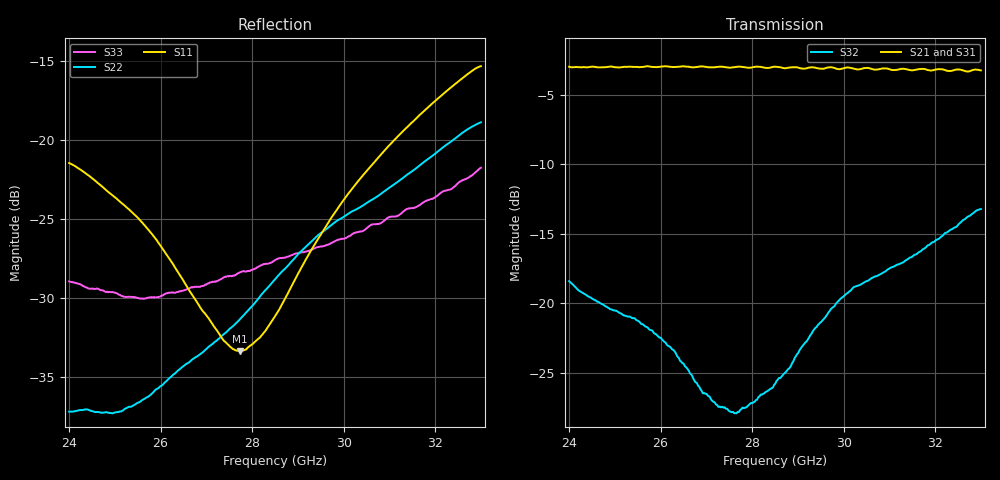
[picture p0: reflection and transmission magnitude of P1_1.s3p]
!The following data was pulled from an Agilent PNA
!This sNp file was generated from the data in the RF Test software
!NOTE:  Smoothing/Math/Corrections applied on any given trace ARE included in the data saved here
# MHz S dB R 50
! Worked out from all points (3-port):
!   1601 points, 24 GHz to 33 GHz, reference 50 ohm
!   strongest paths, dB at 24 GHz, 26.25 GHz, 28.5 GHz, 30.75 GHz, 33 GHz:
!     S21: -3.0, -3.0, -3.0, -3.2, -3.2
!     S31: -3.0, -3.0, -3.1, -3.1, -3.2
!     S32: -18.4, -23.3, -25.8, -18.0, -13.2
!   lowest |S11| = -33.4 dB at 27.73 GHz (marker M1), VSWR 1.04, Z = 50.7 + j2.03 ohm
!   |S11| at or under -10 dB: start of sweep to end of sweep
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24000  -21.47 30.3  -3.09 152.5  -3.09 153.2
       -2.98 152.6  -37.20 147.5  -18.42 104.1
       -2.98 152.8  -18.42 103.7  -28.96 -136.6
25389.38  -24.63 25.4  -3.06 138.7  -3.07 139.4
          -2.99 138.9  -36.84 142.4  -21.10 83.3
          -3.01 139.5  -21.08 83.0  -29.95 -135.6
26266.88  -27.85 26.9  -3.06 130.0  -3.07 130.7
          -3.00 129.9  -34.88 144.1  -23.34 56.8
          -2.98 130.6  -23.35 56.5  -29.68 -133.9
27234.38  -32.07 45.8  -3.06 120.1  -3.09 120.8
          -3.00 120.2  -32.68 141.2  -27.33 25.2
          -3.06 120.4  -27.33 24.9  -28.94 -138.5
27729.38  -33.37 69.1  -3.03 114.8  -3.09 115.7
          -2.98 115.0  -31.37 142.1  -27.72 6.5
          -3.11 115.8  -27.74 6.4  -28.40 -144.4
28500  -31.17 106.2  -3.07 106.8  -3.13 107.8
       -2.98 107.0  -28.83 140.4  -25.81 -33.0
       -3.12 107.9  -25.82 -33.1  -27.62 -153.4
29720.62  -24.98 127.6  -3.13 93.8  -3.17 95.1
          -3.02 94.1  -25.42 130.5  -20.43 -79.7
          -3.16 95.3  -20.43 -79.9  -26.55 -172.9
30367.5  -22.44 128.7  -3.16 86.8  -3.18 88.3
         -3.15 87.7  -24.26 124.5  -18.66 -100.1
         -3.12 88.4  -18.67 -100.2  -25.81 175.7
31678.12  -18.39 123.4  -3.24 72.6  -3.20 74.2
          -3.15 73.6  -21.59 117.1  -16.27 -122.0
          -3.18 74.7  -16.28 -122.2  -24.10 151.3
33000  -15.35 115.4  -3.38 58.2  -3.28 59.8
       -3.25 58.7  -18.90 106.9  -13.17 -141.7
       -3.19 60.5  -13.23 -141.8  -21.77 128.1
